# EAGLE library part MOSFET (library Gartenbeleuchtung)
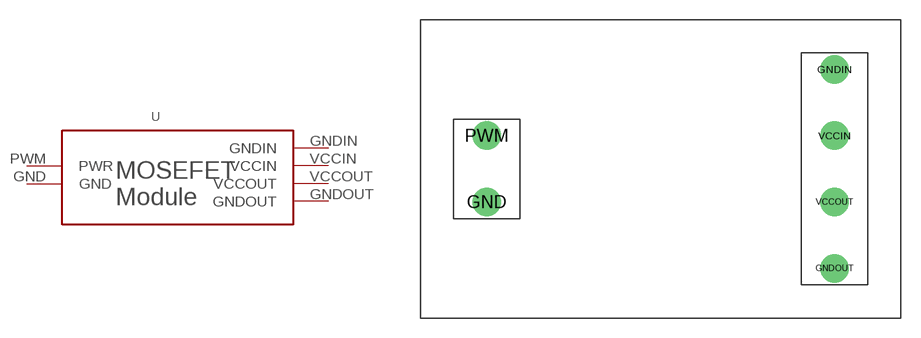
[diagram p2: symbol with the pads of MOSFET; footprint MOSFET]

Designator prefix -

## MOSFET  [MOSFET]
GND  GND  pwr
GNDIN  GNDIN  pwr
GNDOUT  GNDOUT  pwr
PWM  PWR  in
VCCIN  VCCIN  pwr
VCCOUT  VCCOUT  pwr

## Footprint MOSFET (pad centres in mm)
drill 1 pad 2.184: GND -19.05,-5.08; GNDIN 7.62,5.08; GNDOUT 7.62,-10.16; PWM -19.05,0; VCCIN 7.62,0; VCCOUT 7.62,-5.08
